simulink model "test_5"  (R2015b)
settings: Solver=FixedStepDiscrete  StartTime=0.0  StopTime=1  RelTol=1e-3
undefined symbols (not defined in the file or in its folder): fir1

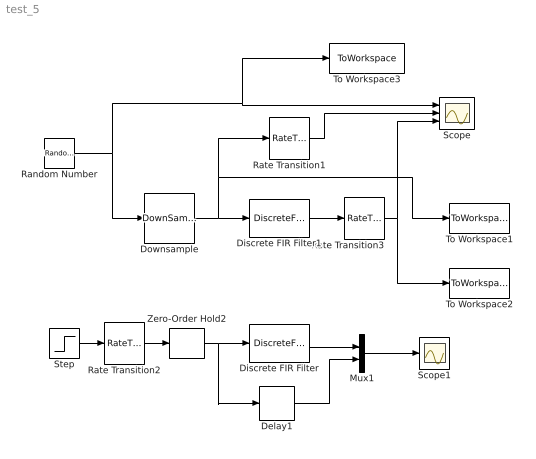
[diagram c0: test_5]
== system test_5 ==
  Delay1 : Delay  DelayLength=8
  Discrete FIR Filter : DiscreteFir  Coefficients=fir1(16,0.01)
  Discrete FIR Filter1 : DiscreteFir  Coefficients=fir1(16,0.5)
  Downsample : DownSample  N=4  RateOptions=Allow multirate processing
  Mux1 : Mux  Inputs=2
  Random Number : RandomNumber  SampleTime=.01
  Rate Transition1 : RateTransition
  Rate Transition2 : RateTransition
  Rate Transition3 : RateTransition
  Scope : Scope  NumInputPorts=3
  Scope1 : Scope
  Step : Step  Time=0.2  SampleTime=.01
  To Workspace1 : ToWorkspace  VariableName=y2  SaveFormat=Timeseries  SampleTime=-1
  To Workspace2 : ToWorkspace  VariableName=y3  SaveFormat=Timeseries  SampleTime=-1
  To Workspace3 : ToWorkspace  VariableName=y1  SaveFormat=Timeseries  SampleTime=-1
  Zero-Order Hold2 : ZeroOrderHold  SampleTime=0.005
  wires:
  Random Number/1 -> Scope/1, To Workspace3/1, Downsample/1
  Discrete FIR Filter/1 -> Mux1/1
  Mux1/1 -> Scope1/1
  Delay1/1 -> Mux1/2
  Step/1 -> Rate Transition2/1
  Discrete FIR Filter1/1 -> Rate Transition3/1
  Rate Transition1/1 -> Scope/2
  Zero-Order Hold2/1 -> Delay1/1, Discrete FIR Filter/1
  Downsample/1 -> Discrete FIR Filter1/1, To Workspace1/1, Rate Transition1/1
  Rate Transition2/1 -> Zero-Order Hold2/1
  Rate Transition3/1 -> Scope/3, To Workspace2/1
